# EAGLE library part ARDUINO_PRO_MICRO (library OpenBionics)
Breakout Board for arduino micro pro.
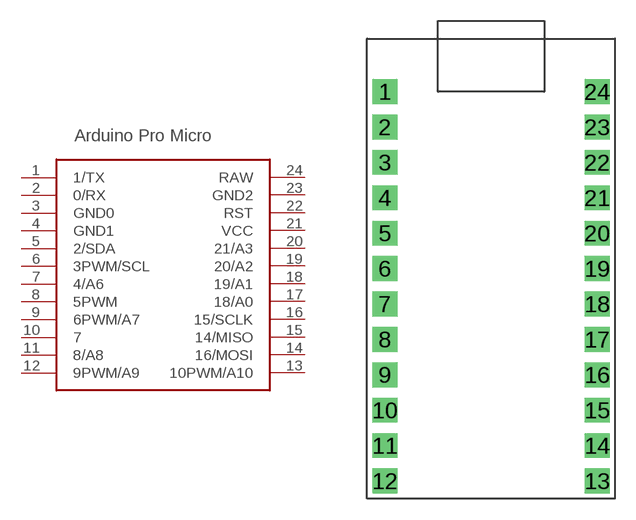
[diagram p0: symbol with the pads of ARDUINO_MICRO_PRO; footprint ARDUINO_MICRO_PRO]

Designator prefix -

## ARDUINO_PRO_MICROARDUINO_BOARD  [ARDUINO_MICRO_PRO]
1  1/TX
2  0/RX
3  GND0
4  GND1
5  2/SDA
6  3PWM/SCL
7  4/A6
8  5PWM
9  6PWM/A7
10  7
11  8/A8
12  9PWM/A9
13  10PWM/A10
14  16/MOSI
15  14/MISO
16  15/SCLK
17  18/A0
18  19/A1
19  20/A2
20  21/A3
21  VCC
22  RST
23  GND2
24  RAW

## Footprint ARDUINO_MICRO_PRO (pad centres in mm)
drill 1 pad 1.778 square: 1 -7.62,12.7; 2 -7.62,10.16; 3 -7.62,7.62; 4 -7.62,5.08; 5 -7.62,2.54; 6 -7.62,0; 7 -7.62,-2.54; 8 -7.62,-5.08; 9 -7.62,-7.62; 10 -7.62,-10.16; 11 -7.62,-12.7; 12 -7.62,-15.24; 13 7.62,-15.24; 14 7.62,-12.7; 15 7.62,-10.16; 16 7.62,-7.62; 17 7.62,-5.08; 18 7.62,-2.54; 19 7.62,0; 20 7.62,2.54; 21 7.62,5.08; 22 7.62,7.62; 23 7.62,10.16; 24 7.62,12.7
